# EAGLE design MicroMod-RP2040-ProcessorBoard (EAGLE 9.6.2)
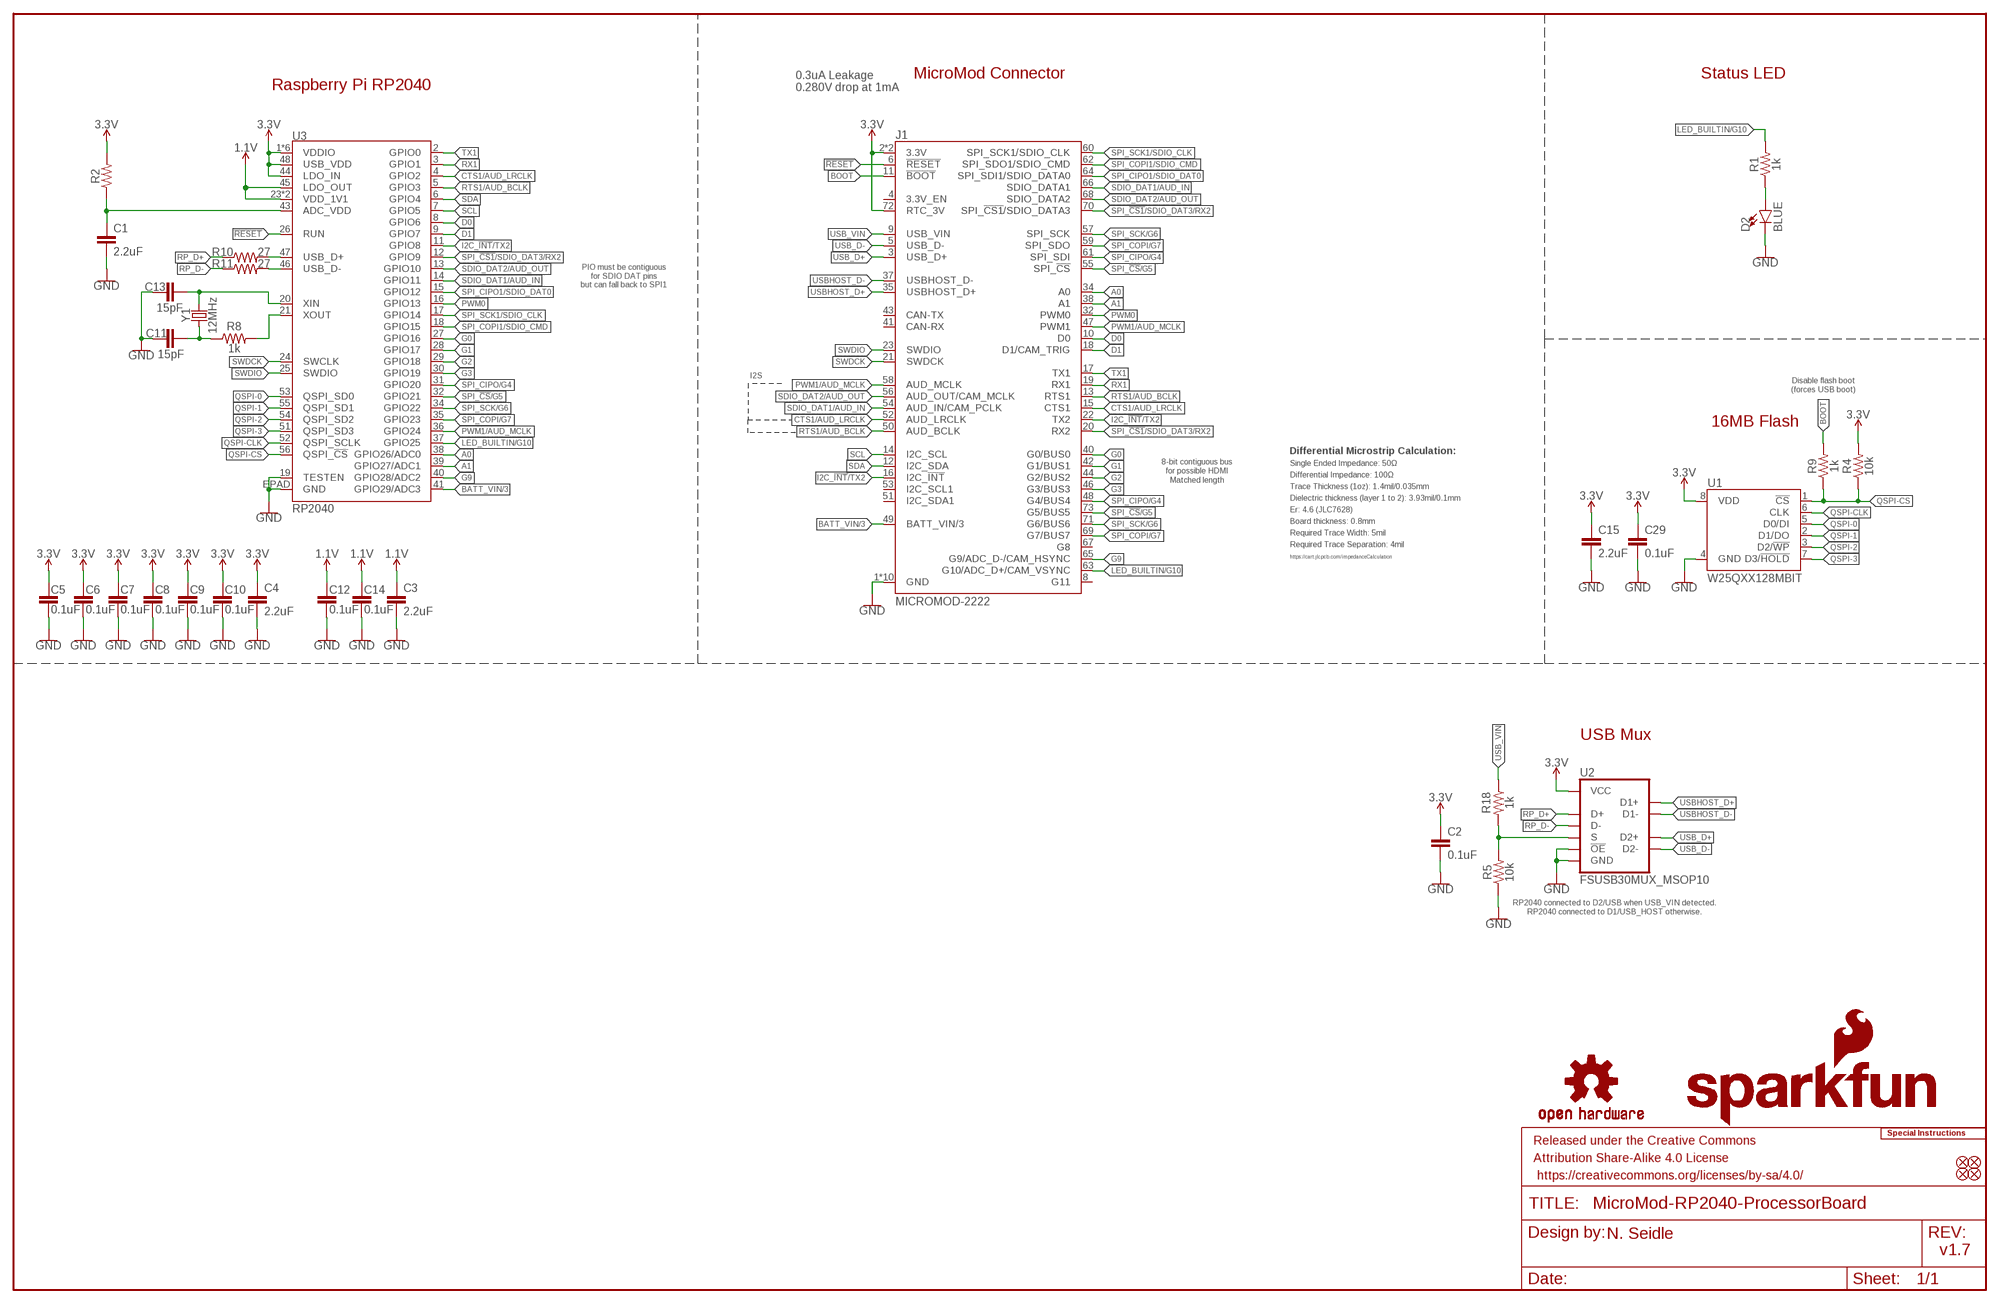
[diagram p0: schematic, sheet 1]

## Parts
C1  2.2uF  2.2UF-0402_TIGHT-10V-10%-X5R  [0402-TIGHT]
C2  0.1uF  0.1UF-0402T-6.3V-10%-X7R  [0402-TIGHT]
C3  2.2uF  2.2UF-0402_TIGHT-10V-10%-X5R  [0402-TIGHT]
C4  2.2uF  2.2UF-0402_TIGHT-10V-10%-X5R  [0402-TIGHT]
C5  0.1uF  0.1UF-0402T-6.3V-10%-X7R  [0402-TIGHT]
C6  0.1uF  0.1UF-0402T-6.3V-10%-X7R  [0402-TIGHT]
C7  0.1uF  0.1UF-0402T-6.3V-10%-X7R  [0402-TIGHT]
C8  0.1uF  0.1UF-0402T-6.3V-10%-X7R  [0402-TIGHT]
C9  0.1uF  0.1UF-0402T-6.3V-10%-X7R  [0402-TIGHT]
C10  0.1uF  0.1UF-0402T-6.3V-10%-X7R  [0402-TIGHT]
C11  15pF  15PF-0402T-50V-5%  [0402-TIGHT]
C12  0.1uF  0.1UF-0402T-6.3V-10%-X7R  [0402-TIGHT]
C13  15pF  15PF-0402T-50V-5%  [0402-TIGHT]
C14  0.1uF  0.1UF-0402T-6.3V-10%-X7R  [0402-TIGHT]
C15  2.2uF  2.2UF-0402_TIGHT-10V-10%-X5R  [0402-TIGHT]
C29  0.1uF  0.1UF-0402T-6.3V-10%-X7R  [0402-TIGHT]
D2  BLUE  LED-BLUE0603  [LED-0603]
FD1  FIDUCIALUFIDUCIAL  [FIDUCIAL-MICRO]
FD2  FIDUCIALUFIDUCIAL  [FIDUCIAL-MICRO]
FD3  FIDUCIALUFIDUCIAL  [FIDUCIAL-MICRO]
FD4  FIDUCIALUFIDUCIAL  [FIDUCIAL-MICRO]
FRAME1  FRAME-LEDGER  [CREATIVE_COMMONS]
J1  MICROMOD-2222  [M.2-CARD-E-22]
LOGO1  SFE_LOGO_NAME_FLAME.1_INCH  [SFE_LOGO_NAME_FLAME_.1]
LOGO2  SFE_LOGO_FLAME.1_INCH  [SFE_LOGO_FLAME_.1]
LOGO3  OSHW-LOGOMINI  [OSHW-LOGO-MINI]
LOGO4  SPECIAL_INSTRUCTIONS-ORDERING  [ORDERING_INSTRUCTIONS]
R1  1k  1KOHM-0402T-1/16W-1%  [0402-TIGHT]
R2  200OHM-0402T-1/16W-1%  [0402-TIGHT]
R4  10k  10KOHM-0402T-1/16W-1%  [0402-TIGHT]
R5  10k  10KOHM-0402T-1/16W-1%  [0402-TIGHT]
R8  1k  1KOHM-0402T-1/16W-1%  [0402-TIGHT]
R9  1k  1KOHM-0402T-1/16W-1%  [0402-TIGHT]
R10  27  27OHM  [0402-TIGHT]
R11  27  27OHM  [0402-TIGHT]
R18  1k  1KOHM-0402T-1/16W-1%  [0402-TIGHT]
U1  W25QXX128MBIT  W25QXX128MBIT-6X5-SKINNY_CENTER  [WSON-8-6X5-SKINNY_CENTERPAD]
U2  FSUSB30MUX_MSOP10  [MSOP10]
U3  RP2040  [QFN-56]
Y1  12MHz  CRYSTAL-12MHZ  [CRYSTAL-SMD-2X2.5MM]

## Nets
1.1V: C3.1 C12.1 C14.1 U3.23(VDD_1V1) U3.45(LDO_OUT) U3.50(VDD_1V1)
3.3V: C2.1 C4.1 C5.1 C6.1 C7.1 C8.1 C9.1 C10.1 C15.1 C29.1 J1.2(3.3V) J1.72(RTC_3V) J1.74(3.3V) R2.2 R4.2 U1.8(VDD) U2.10(VCC) U3.1(VDDIO) U3.10(VDDIO) U3.22(VDDIO) U3.33(VDDIO) U3.42(VDDIO) U3.44(LDO_IN) U3.48(USB_VDD) U3.49(VDDIO)
!RESET!: J1.6(!RESET!) U3.26(RUN)
A0: J1.34(A0) U3.38(GPIO26/ADC0)
A1: J1.38(A1) U3.39(GPIO27/ADC1)
ADC_VDD: C1.1 R2.1 U3.43(ADC_VDD)
BATT_VIN/3: J1.49(BATT_VIN/3) U3.41(GPIO29/ADC3)
BOOT: J1.11(!BOOT!) R9.2
CTS1/AUD_LRCLK: J1.15(CTS1) J1.52(AUD_LRCLK) U3.4(GPIO2)
D0: J1.10(D0) U3.8(GPIO6)
D1: J1.18(D1/CAM_TRIG) U3.9(GPIO7)
G0 [DiffPair]: J1.40(G0/BUS0) U3.27(GPIO16)
G1 [DiffPair]: J1.42(G1/BUS1) U3.28(GPIO17)
G2 [DiffPair]: J1.44(G2/BUS2) U3.29(GPIO18)
G3 [DiffPair]: J1.46(G3/BUS3) U3.30(GPIO19)
G9: J1.65(G9/ADC_D-/CAM_HSYNC) U3.40(GPIO28/ADC2)
GND: C1.2 C2.2 C3.2 C4.2 C5.2 C6.2 C7.2 C8.2 C9.2 C10.2 C11.1 C12.2 C13.1 C14.2 C15.2 C29.2 D2.C J1.1(GND) J1.7(GND) J1.33(GND) J1.36(GND) J1.39(GND) J1.45(GND) J1.75(GND) J1.GND1(GND) J1.GND2(GND) J1.GND3(GND) R5.1 U1.4(GND) U2.5(GND) U2.9(!OE!) U3.19(TESTEN) U3.EPAD(GND)
I2C_!INT!/TX2: J1.16(I2C_!INT!) J1.22(TX2) U3.11(GPIO8)
LED_BUILTIN/G10: J1.63(G10/ADC_D+/CAM_VSYNC) R1.2 U3.37(GPIO25)
N$2: D2.A R1.1
N$4: R8.2 U3.21(XOUT)
N$5: C13.2 U3.20(XIN) Y1.P3
N$6: C11.2 R8.1 Y1.P1
PWM0: J1.32(PWM0) U3.16(GPIO13)
PWM1/AUD_MCLK: J1.47(PWM1) J1.58(AUD_MCLK) U3.36(GPIO24)
QSPI-0: U1.5(D0/DI) U3.53(QSPI_SD0)
QSPI-1: U1.2(D1/DO) U3.55(QSPI_SD1)
QSPI-2: U1.3(D2/!WP!) U3.54(QSPI_SD2)
QSPI-3: U1.7(D3/!HOLD!) U3.51(QSPI_SD3)
QSPI-CLK [Clock]: U1.6(CLK) U3.52(QSPI_SCLK)
QSPI-CS: R4.1 R9.1 U1.1(!CS!) U3.56(QSPI_!CS!)
RP_D1+: R10.2 U3.47(USB_D+)
RP_D1-: R11.2 U3.46(USB_D-)
RP_D+: R10.1 U2.4(D+)
RP_D-: R11.1 U2.6(D-)
RTS1/AUD_BCLK: J1.13(RTS1) J1.50(AUD_BCLK) U3.5(GPIO3)
RX1: J1.19(RX1) U3.3(GPIO1)
SCL: J1.14(I2C_SCL) U3.7(GPIO5)
SDA: J1.12(I2C_SDA) U3.6(GPIO4)
SDIO_DAT1/AUD_IN: J1.54(AUD_IN/CAM_PCLK) J1.66(SDIO_DATA1) U3.14(GPIO11)
SDIO_DAT2/AUD_OUT: J1.56(AUD_OUT/CAM_MCLK) J1.68(SDIO_DATA2) U3.13(GPIO10)
SPI_!CS1!/SDIO_DAT3/RX2: J1.20(RX2) J1.70(SPI_!CS1!/SDIO_DATA3) U3.12(GPIO9)
SPI_!CS!/G5 [DiffPair]: J1.55(SPI_!CS!) J1.73(G5/BUS5) U3.32(GPIO21)
SPI_CIPO1/SDIO_DAT0: J1.64(SPI_SDI1/SDIO_DATA0) U3.15(GPIO12)
SPI_CIPO/G4 [DiffPair]: J1.48(G4/BUS4) J1.61(SPI_SDI) U3.31(GPIO20)
SPI_COPI1/SDIO_CMD: J1.62(SPI_SDO1/SDIO_CMD) U3.18(GPIO15)
SPI_COPI/G7 [DiffPair]: J1.59(SPI_SDO) J1.69(G7/BUS7) U3.35(GPIO23)
SPI_SCK1/SDIO_CLK: J1.60(SPI_SCK1/SDIO_CLK) U3.17(GPIO14)
SPI_SCK/G6 [DiffPair]: J1.57(SPI_SCK) J1.71(G6/BUS6) U3.34(GPIO22)
SWDCK: J1.21(SWDCK) U3.24(SWCLK)
SWDIO: J1.23(SWDIO) U3.25(SWDIO)
TX1: J1.17(TX1) U3.2(GPIO0)
USB_D+: J1.3(USB_D+) U2.3(D2+)
USB_D-: J1.5(USB_D-) U2.7(D2-)
USB_MUX_SIG: R5.2 R18.2 U2.1(S)
USB_VIN: J1.9(USB_VIN) R18.1
USBHOST_D+: J1.35(USBHOST_D+) U2.2(D1+)
USBHOST_D-: J1.37(USBHOST_D-) U2.8(D1-)
Unconnected: J1.4(3.3V_EN) J1.8(G11) J1.41(CAN-RX) J1.43(CAN-TX) J1.51(I2C_SDA1) J1.53(I2C_SCL1) J1.67(G8)

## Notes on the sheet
- MicroMod Connector | Status LED
- Raspberry Pi RP2040
- 0.3uA Leakage
  0.280V drop at 1mA
- PIO must be contiguous
  for SDIO DAT pins
  but can fall back to SPI1
- I2S
- Disable flash boot
  (forces USB boot)
- 16MB Flash
- Differential Microstrip Calculation:
- 8-bit contiguous bus
  for possible HDMI
- Single Ended Impedance: 50Ω
- Differential Impedance: 100Ω
- Matched length
- Trace Thickness (1oz): 1.4mil/0.035mm
- Dielectric thickness (layer 1 to 2): 3.93mil/0.1mm
- Er: 4.6 (JLC7628)
- Board thickness: 0.8mm
- Required Trace Width: 5mil
- Required Trace Separation: 4mil
- https://cart.jlcpcb.com/impedanceCalculation
- USB Mux
- RP2040 connected to D2/USB when USB_VIN detected.
  RP2040 connected to D1/USB_HOST otherwise.
- N. Seidle
- v1.7

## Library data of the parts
C1 C3 C4 C15 = SparkFun-Capacitors:2.2UF: 2.2µF ceramic capacitors; PROD_ID: CAP-14232
C2 C5-C10 C12 C14 C29 = SparkFun-Capacitors:0.1UF: 0.1µF ceramic capacitors; PROD_ID: CAP-14993
C11 C13 = SparkFun-Capacitors:15PF: 15pF ceramic capacitors; PROD_ID: CAP-13063
D2 = SparkFun-LED:LED-BLUE: Blue SMD LED; PROD_ID: DIO-08575
FD1-FD4 = SparkFun-Aesthetics:FIDUCIAL: Fiducial Alignment Points
FRAME1 = SparkFun-Aesthetics:FRAME-LEDGER: Schematic Frame - Ledger
J1 = SparkFun-MicroMod:MICROMOD: MicroMod Connector Description: A card edge connector and mating PCB connector to allow various MicroMod Processor Boards to be coupled with various carrier boards of different capabilities. Based on the M.2 standard.
LOGO1 = SparkFun-Aesthetics:SFE_LOGO_NAME_FLAME: SparkFun Font Logo w/ Flame
LOGO2 = SparkFun-Aesthetics:SFE_LOGO_FLAME: SparkFun Flame Logo
LOGO3 = SparkFun-Aesthetics:OSHW-LOGO: Open-Source Hardware (OSHW) Logo
LOGO4 = SparkFun-Aesthetics:SPECIAL_INSTRUCTIONS: Special Ordering/Production Instructions Alert
R1 R8 R9 R18 = SparkFun-Resistors:1KOHM: 1kΩ resistor; PROD_ID: RES-14342
R2 = SparkFun-Resistors:200OHM: 200Ω resistor; PROD_ID: RES-15550
R4 R5 = SparkFun-Resistors:10KOHM: 10kΩ resistor; PROD_ID: RES-14241
R10 R11 = SparkFun-Resistors:27OHM: 27Ω resistor; PROD_ID: RES-15238
U1 = SparkFun-IC-Memory:W25QXX; PROD_ID: IC-15107
U2 = SparkFun-IC-Special-Function:FSUSB30MUX; PROD_ID: IC-15569
U3 = RP2040:RP2040: Raspberry Pi RP2040 MCU 56-pin 32-bit Microcontroller with 264kB of SRAM and external flash support up to 16MB Getting Started with the RP2040 Dual-core ARM Cortex M0+ processor, flexible clock running up to 133 MHz 264kB of SRAM, and QSPI control of common flash memory USB 1.1 Host and Device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; PROD_ID: IC-15502
Y1 = SparkFun-Clocks:CRYSTAL-12MHZ: 12.0MHz Crystal; PROD_ID: XTAL-15540

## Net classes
1 DiffPair: width 0.127 mm, clearance 0.178 mm
2 Clock: width 0.089 mm, clearance 0.178 mm
4 InternalPower: width 0.152 mm

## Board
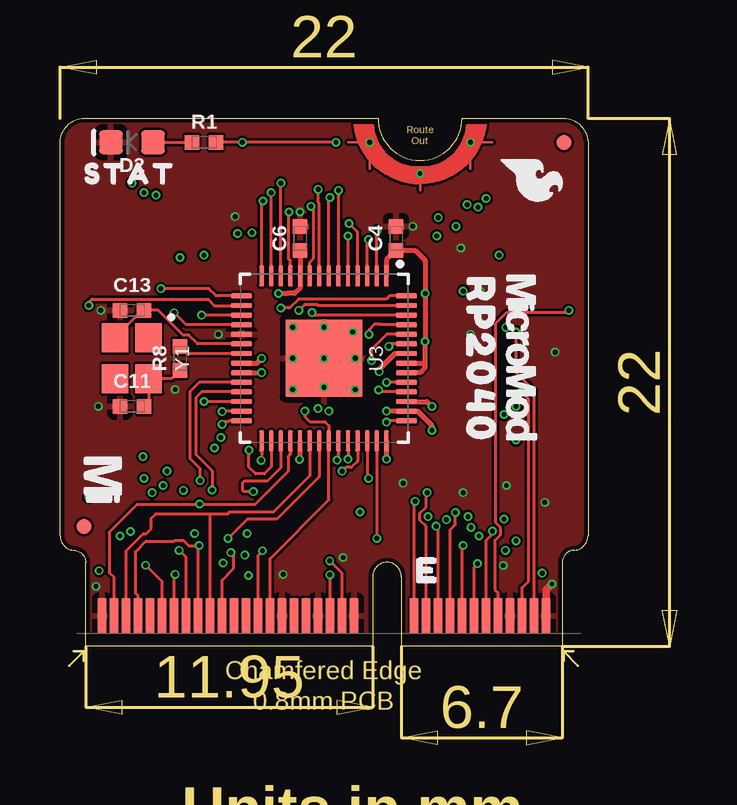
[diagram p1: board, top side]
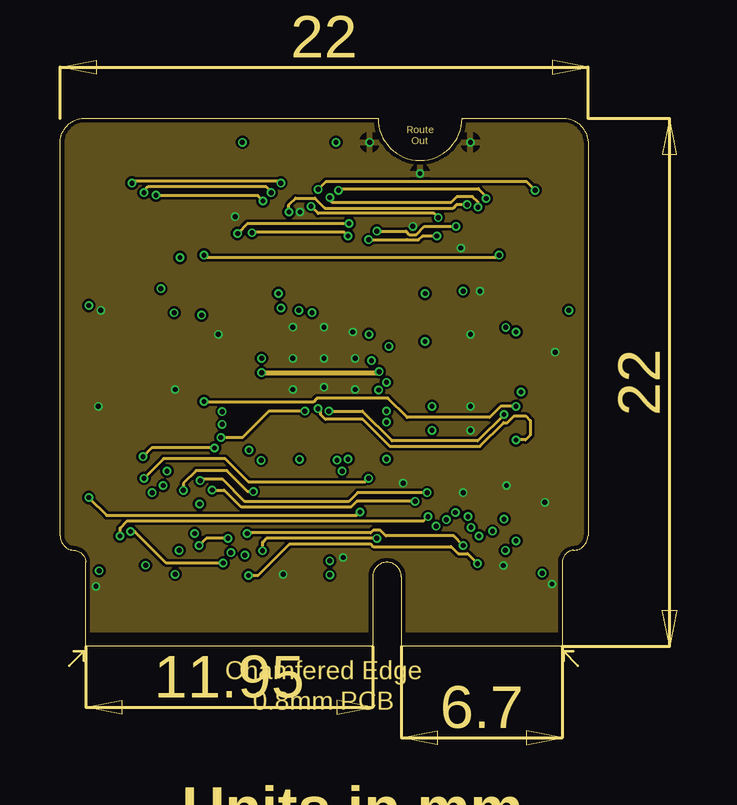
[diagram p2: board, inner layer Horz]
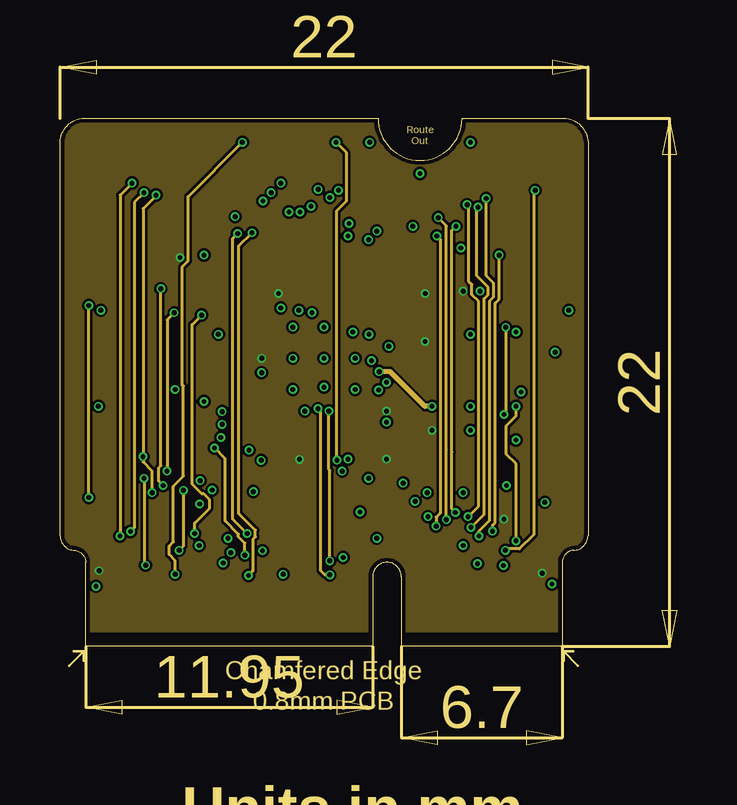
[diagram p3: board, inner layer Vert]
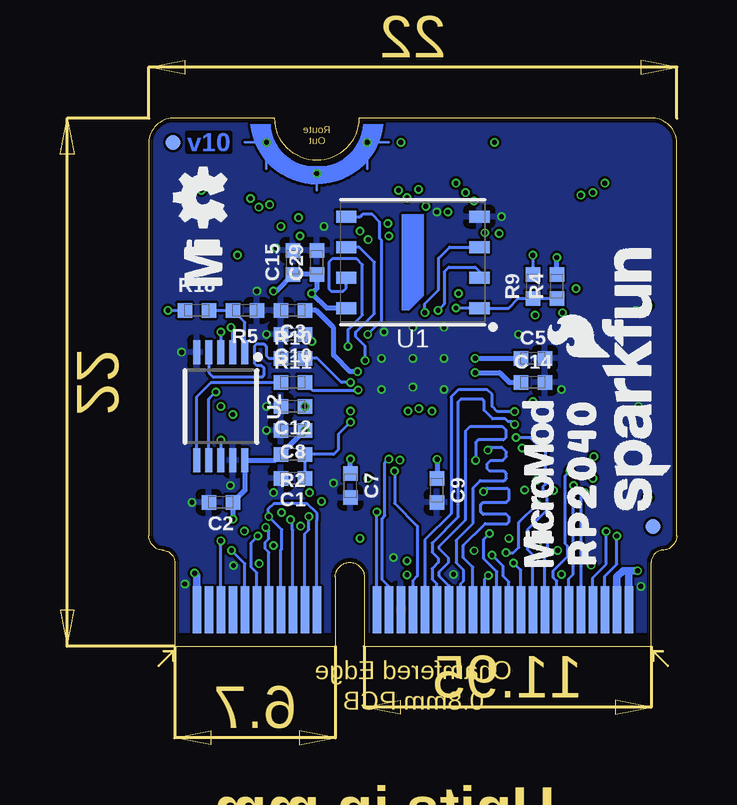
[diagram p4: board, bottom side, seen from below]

Size 25.7 x 28.54 mm. Coordinates in mm from the lower left corner, seen from the top.
Outline: 0,8.71 0,25.11 arc-87 1,26.11 13.25,26.11 arc180 16.75,26.11 21,26.11 arc-87 22,25.11 22,8.71
Outline: 0,8.71 arc87 0.6,8.11
Outline: 21.4,8.11 arc87 22,8.71
Outline: 21.4,8.11 arc85 20.93,7.61 20.93,4.11 14.22,4.11 14.22,7.01 arc180 13.03,7.01 13.03,4.11 1.07,4.11 1.07,7.61 arc84 0.6,8.11
Outline: 21.4,8.11 arc87 22,8.71
Outline: 0,8.71 arc87 0.6,8.11
Copper layers (1+2*15+16): Top 0.035mm / dielectric 1.5mm / Horz 0.035mm / dielectric 0.15mm / Vert 0.035mm / dielectric 0.2mm / Bottom 0.035mm
Design rules "SparkFun-4-layer-MicroMod": minimum track width 4mil, minimum drill 0.2mm, track to track 4mil, track to pad 4mil, pad to pad 4mil, via to via 4mil, smd to smd 4mil, copper to edge 6mil, drill to drill 6mil, minimum pad ring 3mil, minimum via ring 3mil, stop-mask expansion 4mil, vias tented up to drill 25mil, thermal gap 10mil

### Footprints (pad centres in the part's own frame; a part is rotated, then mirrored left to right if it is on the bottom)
0402-TIGHT = smd 0.6 x 0.6: 1 -0.5,0; 2 0.5,0
LED-0603 = smd 1 x 1: A -0.877,0; C 0.877,0
FIDUCIAL-MICRO = smd 0.635 x 0.635: 1 0,0
M.2-CARD-E-22 = smd 0.35 x 1.45: 1 9.25,1.275; 3 8.75,1.275; 5 8.25,1.275; 7 7.75,1.275; 9 7.25,1.275; 11 6.75,1.275; 13 6.25,1.275; 15 5.75,1.275; 17 5.25,1.275; 19 4.75,1.275; 21 4.25,1.275; 23 3.75,1.275; 33 1.25,1.275; 35 0.75,1.275; 37 0.25,1.275; 39 -0.25,1.275; 41 -0.75,1.275; 43 -1.25,1.275; 45 -1.75,1.275; 47 -2.25,1.275; 49 -2.75,1.275; 51 -3.25,1.275; 53 -3.75,1.275; 55 -4.25,1.275; 57 -4.75,1.275; 59 -5.25,1.275; 61 -5.75,1.275; 63 -6.25,1.275; 65 -6.75,1.275; 67 -7.25,1.275; 69 -7.75,1.275; 71 -8.25,1.275; 73 -8.75,1.275; 75 -9.25,1.275 | smd 0.35 x 1.95 bottom: 2 9,1.525; 4 8.5,1.525; 6 8,1.525; 8 7.5,1.525; 10 7,1.525; 12 6.5,1.525; 14 6,1.525; 16 5.5,1.525; 18 5,1.525; 20 4.5,1.525; 22 4,1.525; 32 1.5,1.525; 34 1,1.525; 36 0.5,1.525; 38 0,1.525; 40 -0.5,1.525; 42 -1,1.525; 44 -1.5,1.525; 46 -2,1.525; 48 -2.5,1.525; 50 -3,1.525; 52 -3.5,1.525; 54 -4,1.525; 56 -4.5,1.525; 58 -5,1.525; 60 -5.5,1.525; 62 -6,1.525; 64 -6.5,1.525; 66 -7,1.525; 68 -7.5,1.525; 70 -8,1.525; 72 -8.5,1.525; 74 -9,1.525 | drill 0.2: GND1 1.9,21; GND2 4,19.7; GND3 6.1,21
WSON-8-6X5-SKINNY_CENTERPAD = smd 0.85 x 0.5: 1 -2.775,1.905; 2 -2.775,0.635; 3 -2.775,-0.635; 4 -2.775,-1.905; 5 2.775,-1.905; 6 2.775,-0.635; 7 2.775,0.635; 8 2.775,1.905
MSOP10 = smd 1 x 0.3: 1 -2.25,1; 2 -2.25,0.5; 3 -2.25,0; 4 -2.25,-0.5; 5 -2.25,-1; 6 2.25,-1; 7 2.25,-0.5; 8 2.25,0; 9 2.25,0.5; 10 2.25,1
QFN-56 = smd 0.875 x 0.2: 1 -3.437,2.6; 2 -3.437,2.2; 3 -3.437,1.8; 4 -3.437,1.4; 5 -3.437,1; 6 -3.437,0.6; 7 -3.437,0.2; 8 -3.437,-0.2; 9 -3.437,-0.6; 10 -3.437,-1; 11 -3.437,-1.4; 12 -3.437,-1.8; 13 -3.437,-2.2; 14 -3.437,-2.6; 29 3.437,-2.6; 30 3.437,-2.2; 31 3.437,-1.8; 32 3.437,-1.4; 33 3.437,-1; 34 3.437,-0.6; 35 3.437,-0.2; 36 3.437,0.2; 37 3.437,0.6; 38 3.437,1; 39 3.437,1.4; 40 3.437,1.8; 41 3.437,2.2; 42 3.437,2.6 | smd 0.2 x 0.875: 15 -2.6,-3.437; 16 -2.2,-3.437; 17 -1.8,-3.437; 18 -1.4,-3.437; 19 -1,-3.437; 20 -0.6,-3.437; 21 -0.2,-3.437; 22 0.2,-3.437; 23 0.6,-3.437; 24 1,-3.437; 25 1.4,-3.437; 26 1.8,-3.437; 27 2.2,-3.437; 28 2.6,-3.437; 43 2.6,3.437; 44 2.2,3.437; 45 1.8,3.437; 46 1.4,3.437; 47 1,3.437; 48 0.6,3.437; 49 0.2,3.437; 50 -0.2,3.437; 51 -0.6,3.437; 52 -1,3.437; 53 -1.4,3.437; 54 -1.8,3.437; 55 -2.2,3.437; 56 -2.6,3.437 | smd 3.2 x 3.2: EPAD 0,0
CRYSTAL-SMD-2X2.5MM = smd 1.2 x 1.1: P1 0.846,0.69; P2 -0.854,0.69; P3 -0.854,-0.71; P4 0.846,-0.71

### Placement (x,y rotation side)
C1  16,11.11 180 bottom
C2  19,10.11 180 bottom
C3  16,18.11 180 bottom
C4  14,21.11 90 top
C5  6,16.11 0 bottom
C6  10,21.11 90 top
C7  13.6,10.81 270 bottom
C8  16,13.11 180 bottom
C9  10,10.61 270 bottom
C10  16,17.11 180 bottom
C11  3,14.11 0 top
C12  16,14.11 180 bottom
C13  3,18.11 0 top
C14  6,15.11 0 bottom
C15  16,20.11 90 bottom
C29  15,20.11 90 bottom
D2  3,25.11 180 top
FD1  1,9.11 0 top
FD2  21,25.11 0 top
FD3  21,25.11 0 bottom
FD4  1,9.11 0 bottom
FRAME1  not placed on the board
J1  11,4.11 0 top
LOGO1  1.7,15.31 90 bottom
LOGO2  19.68,23.54 270 top
LOGO3  19.75,22.81 90 bottom
LOGO4  not placed on the board
R1  6,25.11 0 top
R2  16,12.11 180 bottom
R4  5,19.11 90 bottom
R5  18,18.11 180 bottom
R8  5,16.11 90 top
R9  6,19.11 90 bottom
R10  16,16.11 0 bottom
R11  16,15.11 0 bottom
R18  20,18.11 0 bottom
U1  11,20.11 180 bottom
U2  19,14.11 270 bottom
U3  11,16.11 270 top
U$1  [MICROMOD_MI_LOGO_.35]  1.81,11.08 270 top
U$3  [MICROMOD_LOGO_.3]  5.71,10.84 90 bottom
U$4  [RP20400]  3.94,10.97 90 bottom
U$7  [MICROMOD_MI_LOGO_.35]  19.75,20.07 90 bottom
U$9  [RP20400]  17.53,16.05 270 top
U$11  [STAT0]  0.38,23.79 0 top
U$12  [MICROMOD_LOGO_.3]  19.18,16.18 270 top
Y1  3,16.11 270 top

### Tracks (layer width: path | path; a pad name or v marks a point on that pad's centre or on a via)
1.1V  (via drill 0.2)
  Top 0.203: U3.45 15.3,14.31 C12.1 | U3.50 13.95,16.31 13.3,15.66 v13.3,15.56 | U3.23 v8.4,15.51
  Horz 0.127: v13.3,15.56 13.3,15.51
  Horz 0.203: v8.4,15.51 13.3,15.51
  Vert 0.203: C12.1 15.2,14.11 13.75,15.56 v13.3,15.56
  Bottom 0.203: v8.4,15.51 7.38,15.51 6.98,15.11 C14.1 | v13.3,15.56 13.62,15.56 14.3,16.23 14.3,17.38 15.03,18.11 C3.1
  other vias: 15.5,14.11
3.3V  (via drill 0.2)
  Top 0.127: v15.21,16.81 v15.21,16.82
  Top 0.203: U3.42 v13.6,11.91 | v13.6,13.91 U3.44 14.9,13.91 15.5,13.31 C8.1 | U3.48 15,15.51 15.21,15.72 15.21,15.91 | v9.98,11.9 10,11.92 U3.33 | C6.1 U3.10 10,19.04 9.77,18.81 9.48,18.81 v9.1,18.81 | U3.1 13.6,20.21 C4.1 14.8,20.61 15.21,20.2 v15.21,18.81 v15.21,16.82 | v15.21,16.81 15.21,15.91 | U3.49 15.21,15.91 | U3.22 8.2,15.91 v8.4,16.11
  Bottom 0.127: v15.21,16.82 v15.21,16.81 | C9.1 9.98,11.13 | 15.18,18.81 v15.21,18.81
  Bottom 0.203: C10.1 v15.21,16.82 | v9.98,11.9 9.98,11.13 | R4.2 v5,20.31 | v18.5,9.41 C2.1 18,10.61 U2.10 16.75,11.86 R2.2 C8.1 | C7.1 v13.6,11.91 | v16.8,18.91 16.7,18.91 C15.1 C29.1 15,19.02 v15.21,18.81 | 15.18,18.81 14.57,18.21 U1.8 | v8.4,16.11 C5.1
  Bottom 0.305: J1.72 2.5,7 2.24,7.26 v1.63,7.26 1.93,7.26 2,7.19 J1.74 | J1.2 20,7.07 v20.09,7.16
  other vias: 15.5,13.11
  pour Vert (isolate 0.102): 0,26.11 22,26.11 22,4.75 0,4.75
!RESET!  (via drill 0.2)
  Top 0.127: U3.26 v6,14.31
  Horz 0.127: v6,14.31 10.56,14.31 10.71,14.45 13.66,14.45 14.46,13.65 17.9,13.65 18.36,14.11 v19,14.11
  Vert 0.127: v19,8.51 19,11.71 18.6,12.11 18.6,13.31 19,13.71 v19,14.11
  Bottom 0.127: J1.6 v19,8.51
A0  (via drill 0.2)
  Top 0.127: U3.38 v12,11.91
  Bottom 0.127: J1.34 12,6.61 12.27,6.88 12.27,9.46 12.16,9.57 12.16,11.75 v12,11.91
A1  (via drill 0.2)
  Top 0.127: v11.76,11.41 11.92,11.57 12.14,11.57 12.4,11.83 U3.39
  Bottom 0.127: v11.76,11.41 11.76,10.07 10.8,9.12 10.8,7.04 11,6.85 J1.38
ADC_VDD  (via drill 0.2)
  Top 0.127: U3.43 13.66,13.51 v13.6,13.45
  Bottom 0.127: v13.6,13.45 14.1,12.95 14.1,12.31 14.3,12.11 R2.1 C1.1
BATT_VIN/3  (via drill 0.2)
  Top 0.127: U3.41 v13.2,8.61 | v8.44,8.09 8.25,7.9 J1.49
  Horz 0.127: v13.2,8.61 8.6,8.61 8.44,8.45 v8.44,8.09
BOOT  (via drill 0.2)
  Top 0.127: J1.11 17.75,8.52 18.02,8.79 v18.02,8.91
  Horz 0.127: v18.3,20.41 18.2,20.31 6.1,20.31 v6,20.41
  Vert 0.127: v18.02,8.91 18.02,9.16 18.13,9.26 18.13,18.41 18.3,18.58 v18.3,20.41
  Bottom 0.127: v6,20.41 R9.2
CTS1/AUD_LRCLK  (via drill 0.2)
  Top 0.127: U3.4 12.4,21.37 v12.04,21.73 | J1.15 16.75,8.26 v16.8,8.31
  Horz 0.127: v12.04,21.73 7.82,21.73 v7.4,21.31 | v16.8,8.31 16.4,8.71 13.58,8.71 13.34,8.95 13.06,8.95 12.95,8.84 7.83,8.84 v7.8,8.81
  Vert 0.127: v7.4,21.31 7.2,21.11 7.2,9.41 v7.8,8.81
  Bottom 0.127: J1.52 7.5,7.23 8.04,7.77 8.04,8.57 v7.8,8.81
D0  (via drill 0.2)
  Top 0.127: U3.8 10.8,22.58 10.76,22.62 v10.76,23.15
  Horz 0.127: v10.76,23.15 11.08,23.47 19.44,23.47 v19.8,23.11
  Vert 0.127: v18.56,8.11 18.61,8.17 19.14,8.17 19.75,8.77 19.75,23.06 v19.8,23.11
  Bottom 0.127: J1.10 18,7.55 v18.56,8.11
D1  (via drill 0.2)
  Top 0.127: U3.9 10.4,20.11 10.57,20.28 10.57,22.33 v10.46,22.44
  Horz 0.127: v10.46,22.44 10.76,22.14 15.59,22.14 v15.76,21.97
  Vert 0.127: v16.09,9.39 16.09,12.3 16.1,12.31 16.1,21.63 v15.76,21.97
  Bottom 0.127: v16.09,9.39 16.01,9.31 16.01,8.97 16,8.96 J1.18
G0  (via drill 0.2)
  Top 0.127: U3.27 6.78,13.91 v6.76,13.89
  Bottom 0.127: J1.40 10.5,8.54 9.4,9.64 9.4,14.5 9.11,14.8 7.9,14.8 7.7,14.61 7.7,14.11 7.48,13.89 v6.76,13.89
G1  (via drill 0.2)
  Top 0.127: U3.28 7.07,13.51 7.03,13.47 6.87,13.47 v6.76,13.36
  Bottom 0.127: v6.76,13.36 6.87,13.47 7.03,13.47 7.14,13.58 7.67,13.58 8.03,13.94 8.03,14.34 8.1,14.41 9,14.41 9.1,14.31 9.1,9.51 10.2,8.41 10.2,8.04 9.93,7.78 9.93,7.61 10.2,7.35 10.2,6.91 10,6.71 J1.42
G2  (via drill 0.2)
  Top 0.127: v8.38,11.86 8.4,11.88 U3.29
  Bottom 0.127: J1.44 9.5,6.64 9.89,7.03 9.89,7.22 9.51,7.61 9.51,7.78 9.89,8.17 9.89,8.29 8.79,9.38 8.79,13.08 8.6,13.28 7.27,13.28 7.12,13.13 7.12,12.81 7.22,12.71 8.27,12.71 8.38,12.59 v8.38,11.86
G3  (via drill 0.2)
  Top 0.127: v7.87,12.28 7.87,11.58 8.15,11.3 8.51,11.3 8.8,11.59 U3.30
  Bottom 0.127: J1.46 9,6.72 8.88,6.84 8.88,7.28 9.2,7.6 9.2,8.53 8.48,9.24 8.48,10.72 8.19,11.01 7.2,11.01 7.1,11.11 7.1,11.31 7.2,11.41 7.8,11.41 7.9,11.51 7.9,11.71 7.75,11.86 7.25,11.86 7.1,12.01 7.1,12.21 7.29,12.41 7.75,12.41 v7.87,12.28
G9  (via drill 0.2)
  Top 0.127: U3.40 12.8,11.17 v12.86,11.11 | J1.65 4.25,6.81 v3.57,7.49
  Horz 0.127: v3.5,11.11 4.32,11.93 6.88,11.93 7.83,10.97 12.72,10.97 v12.86,11.11
  Vert 0.127: v3.5,11.11 3.5,7.56 v3.57,7.49
GND  (via drill 0.2)
  Top 0.305: J1.1 20.25,6.46 v20.5,6.71
  other vias: 18.47,7.48 16.8,10.51 17.1,13.11 18.6,10.81 17.1,14.11 20.63,16.37 16.7,20.71 14.7,21.61 7.3,22.01 6.6,17.11 14.3,10.91 9.7,17.41 12.2,17.21 12.3,14.81 9.7,14.81 11,16.11 1.6,14.11 1.7,18.11 4.8,14.81 17.5,18.91 17.1,17.11 11.8,7.81 9.3,7.11 1.5,6.61 10,22.21 9.7,16.11 12.3,16.11 11,14.91 11,17.41 20.2,10.11
  pour Top (isolate 0.102): 0,26.11 22,26.11 22,4.71 0,4.71
  pour Bottom (isolate 0.102): 0,26.11 22,26.11 22,4.71 0,4.71
  pour Horz (isolate 0.102): 0,4.75 0,26.11 22,26.11 22,4.75
I2C_!INT!/TX2  (via drill 0.2)
  Top 0.127: U3.11 9.6,20.18 9.54,20.24 v9.54,22.2 v9.54,22.21
  Horz 0.127: v9.54,22.21 9.54,22.51 9.82,22.79 10.62,22.79 11.04,22.37 16.38,22.37 16.52,22.51 v16.96,22.51
  Vert 0.127: v17,9.51 17.44,9.95 17.44,18.49 17.16,18.77 17.16,19.19 17.04,19.3 17.04,22.43 v16.96,22.51
  Bottom 0.127: J1.16 16.5,8.13 16.46,8.17 16.46,8.97 v17,9.51 17.04,9.55 17.04,9.81 16.79,10.06 15.4,10.06 14.99,9.65 14.99,9.37 15,9.36 J1.22
LED_BUILTIN/G10  (via drill 0.2)
  Top 0.127: U3.37 11.6,11.92 v11.54,11.86 | v11.5,25.11 v7.6,25.11 R1.2 | J1.63 4.75,7.06 v4.8,7.11
  Vert 0.127: v11.54,11.86 11.54,22.27 11.94,22.67 11.94,24.67 v11.5,25.11 | v4.8,7.11 4.8,7.69 4.55,7.94 4.55,8.28 4.72,8.46 4.72,10.78 5.14,11.2 5.14,14.95 5.1,14.99 5.1,19.93 5.34,20.17 5.34,22.85 v7.6,25.11
N$2
  Top 0.127: D2.A R1.1
N$4
  Top 0.127: U3.21 5.3,16.31 R8.2
N$5
  Top 0.127: Y1.P3 3.44,18.11 C13.2 4.1,18.11 5.13,17.07 5.37,17.07 5.73,16.71 U3.20
N$6
  Top 0.127: R8.1 4.65,15.26 Y1.P1 3.69,14.3 C11.2
PWM0  (via drill 0.2)
  Top 0.127: U3.16 6.43,18.31 6.17,18.57 1.33,18.57 1.2,18.44 v1.2,18.31
  Horz 0.127: v1.2,10.31 1.95,9.56 12.35,9.56 v12.5,9.71
  Vert 0.127: v1.2,10.31 v1.2,18.31
  Bottom 0.127: J1.32 v12.5,9.71
PWM1/AUD_MCLK  (via drill 0.2)
  Top 0.127: J1.47 8.75,7.77 11.2,10.22 U3.36 11.2,13.31 11.04,13.47 10.4,13.47 10.2,13.67 v10.2,13.91
  Horz 0.127: v10.2,13.91 8.7,13.91 7.6,12.81 v6.7,12.81
  Bottom 0.127: v6.7,12.81 6.1,12.81 5.46,12.17 5.46,10.88 5.56,10.78 5.56,10.44 5.4,10.28 5.4,9.8 6.22,8.98 6.22,8.14 6,7.92 J1.58
QSPI-0  (via drill 0.2)
  Top 0.127: U3.53 13.37,17.51 13.36,17.53 13.1,17.53 12.88,17.31 v12.88,17.11
  Bottom 0.127: U1.5 13.2,22.02 13.1,22.11 12.7,22.11 12.38,21.79 12.38,21.11 12.3,21.03 12.3,17.69 v12.88,17.11
QSPI-1  (via drill 0.2)
  Top 0.127: U3.55 10.76,18.31 10.72,18.35 10.2,18.35 v9.95,18.11
  Bottom 0.127: U1.2 8.22,19.73 8.4,19.91 9.5,19.91 9.7,19.71 9.7,18.36 v9.95,18.11
QSPI-2  (via drill 0.2)
  Top 0.127: U3.54 10.6,17.91 v10.5,18.01
  Bottom 0.127: v10.5,18.01 10.5,18.39 9.93,18.96 9.93,20.28 9.46,20.75 U1.3
QSPI-3  (via drill 0.2)
  Top 0.127: U3.51 13.8,16.71 v13.7,16.61
  Bottom 0.127: v13.7,16.61 13.7,17.31 13.1,17.91 13.1,20.01 13.34,20.25 14.36,20.25 14.5,20.11 14.5,19.01 14.4,18.91 13.9,18.91 13.78,19.04 U1.7
QSPI-CLK  (via drill 0.2)
  Top 0.127: U3.52 13.61,17.11 12.98,16.48 v12.98,16.01
  Bottom 0.127: v12.98,16.01 12.98,16.61 13.38,17.01 13.38,17.2 12.61,17.97 12.61,20.11 13.23,20.75 U1.6
QSPI-CS  (via drill 0.2)
  Top 0.127: v9.2,18.21 9.57,18.21 9.94,18.58 13.61,18.58 13.74,18.71 U3.56
  Bottom 0.127: R4.1 R9.1 6.6,18.61 7,18.21 U1.1 v9.2,18.21
RP_D1+  (via drill 0.2)
  Top 0.127: U3.47 v13.6,15.11
  Bottom 0.127: v13.6,15.11 13.98,15.11 14.98,16.11 R10.2
RP_D1-  (via drill 0.2)
  Top 0.127: U3.46 13.36,14.71 v13.28,14.79
  Bottom 0.127: v13.28,14.79 13.44,14.79 13.46,14.77 15.16,14.77 R11.2
RP_D+
  Bottom 0.127: U2.4 19.5,15.51 19.33,15.34 17.27,15.34 17.2,15.41 17.2,15.71 17.3,15.81 17.5,15.81 17.6,15.91 17.6,16.61 17.5,16.71 17.2,16.71 17.1,16.61 17.1,16.21 17,16.11 R10.1
RP_D-
  Bottom 0.127: U2.6 20,14.51 19.4,15.11 R11.1
RTS1/AUD_BCLK  (via drill 0.2)
  Top 0.127: U3.5 v12,21.21 | J1.13 17.25,7.4 v17.4,7.55
  Horz 0.127: v12,21.21 11.84,21.37 8.03,21.37 v8,21.34 | v17.4,7.55 16.98,7.97 16.6,7.97 16.3,8.27 13.06,8.27 12.95,8.38 9.57,8.38 8.26,7.07 v7.86,7.07
  Vert 0.127: v7.86,7.07 8.04,7.25 8.04,8.57 8.14,8.67 8.14,8.95 7.45,9.64 7.45,20.8 v8,21.34
  Bottom 0.127: J1.50 8,6.92 v7.86,7.07
RX1  (via drill 0.2)
  Top 0.127: U3.3 12.8,20.99 v12.86,21.05 | J1.19 15.75,9.04 v15.67,9.12
  Horz 0.127: v15.7,21.21 15.11,21.21 14.94,21.04 14.46,21.04 14.45,21.05 v12.86,21.05
  Vert 0.127: v15.7,21.21 15.84,21.07 15.84,9.66 15.67,9.5 v15.67,9.12
SCL  (via drill 0.2)
  Top 0.127: v11.24,22.81 11.2,22.77 U3.7
  Horz 0.127: v17.42,22.41 17.42,22.62 17.18,22.85 16.54,22.85 16.29,22.6 11.35,22.6 11.24,22.71 v11.24,22.81
  Vert 0.127: v17.13,9.07 17.67,9.61 17.67,18.6 17.84,18.77 17.84,19.07 17.37,19.54 17.37,22.36 v17.42,22.41
  Bottom 0.127: v17.13,9.07 17,8.94 17,8.59 17.14,8.45 17.14,8.17 17,8.03 J1.14
SDA  (via drill 0.2)
  Top 0.127: v11.6,23.11 U3.6
  Horz 0.127: v17.76,22.77 17.76,22.85 17.43,23.18 11.67,23.18 v11.6,23.11
  Vert 0.127: v17.45,8.71 17.45,8.91 17.9,9.36 17.9,18.5 18.07,18.67 18.07,19.24 17.76,19.55 v17.76,22.77
  Bottom 0.127: J1.12 17.5,7.17 17.74,7.41 17.74,8.42 v17.45,8.71
SDIO_DAT1/AUD_IN  (via drill 0.2)
  Top 0.127: U3.14 8.4,22.61 v8.46,22.67
  Horz 0.127: v8.46,22.67 8.24,22.88 4.03,22.88 v4,22.91 | v6.44,12.37 3.82,12.37 v3.46,12.01
  Vert 0.127: v4,22.91 4,22.89 3.46,22.35 v3.46,12.01 3.46,11.79 3.84,11.41 v3.84,10.51 | v7.7,7.91 7.7,8.41 7.43,8.68 7.43,8.79 6.88,9.34 6.88,11.93 v6.44,12.37
  Bottom 0.127: J1.54 7,6.8 7.24,7.04 7.24,7.45 v7.7,7.91 | v3.84,10.51 4,10.35 J1.66
SDIO_DAT2/AUD_OUT  (via drill 0.2)
  Top 0.127: U3.13 v8.8,23.01
  Horz 0.127: v3.5,23.01 3.5,23.09 3.66,23.25 8.6,23.25 8.8,23.05 v8.8,23.01 | v2.94,8.89 3.12,8.89 4.43,7.58 v6.8,7.58
  Vert 0.127: v3.5,23.01 3.1,22.61 3.1,9.05 v2.94,8.89
  Bottom 0.127: J1.68 3.5,6.97 2.94,7.53 v2.94,8.89 | J1.56 6.5,7.28 v6.8,7.58
SPI_!CS1!/SDIO_DAT3/RX2  (via drill 0.2)
  Top 0.127: U3.12 v9.2,23.41
  Horz 0.127: v9.2,23.41 9.16,23.41 9.09,23.48 3.06,23.48 v3,23.42 v3,23.41 | v15.33,9.51 15.15,9.33 2.8,9.33 2.5,9.03 v2.5,8.71
  Vert 0.127: v3,23.41 2.5,22.91 v2.5,8.71
  Bottom 0.127: J1.70 3,7.04 2.5,7.54 v2.5,8.71 | J1.20 15.5,8.8 15.33,8.97 v15.33,9.51
SPI_!CS!/G5  (via drill 0.2)
  Top 0.127: J1.73 2.25,6.99 2.05,7.19 2.05,8.86 3.2,10.01 5.82,10.01 v5.82,10.04 5.84,10.02 8.11,10.02 9.51,11.41 9.51,12.02 9.6,12.11 U3.32 | J1.55 6.75,6.87 7.22,7.34 7.22,7.91 v7.12,8.01
  Bottom 0.127: v5.82,10.04 6.58,9.27 6.58,8.24 6.8,8.01 v7.12,8.01
SPI_CIPO1/SDIO_DAT0  (via drill 0.2)
  Top 0.127: U3.15 6.5,18.71 6.2,19.01 v4.2,19.01
  Vert 0.127: v4.2,19.01 4.2,11.63 4.12,11.55 4.12,10.99 v4.3,10.81
  Bottom 0.127: J1.64 4.5,6.93 4.32,7.11 4.32,10.79 v4.3,10.81
SPI_CIPO/G4  (via drill 0.2)
  Top 0.127: J1.61 5.25,7.83 v4.96,8.11 | U3.31 9.2,11.55 8.64,10.99 7.68,10.99 7.6,10.91 7.6,10.61 7.66,10.55 v8.05,10.55
  Horz 0.127: v8.05,10.55 7.82,10.55 6.95,11.43 5.67,11.43 5.14,10.9 v5.14,10.61
  Vert 0.127: v5.14,10.61 5.14,8.29 v4.96,8.11
  Bottom 0.127: J1.48 8.5,7.41 8.89,7.8 8.89,8.32 7.98,9.23 7.07,9.23 6.99,9.31 6.99,9.5 7.1,9.61 8.08,9.61 8.18,9.71 8.18,10.01 8.08,10.11 7.1,10.11 6.99,10.22 6.99,10.61 7.08,10.71 7.91,10.71 v8.05,10.55
SPI_COPI1/SDIO_CMD  (via drill 0.2)
  Top 0.127: U3.18 5.26,17.51 v4.76,18.01
  Vert 0.127: v4.76,18.01 4.46,17.71 v4.46,11.41
  Bottom 0.127: v4.46,11.41 4.64,11.23 4.64,8.38 4.55,8.28 4.55,7.86 5.14,7.27 5.14,6.97 5,6.83 J1.62
SPI_COPI/G7  (via drill 0.2)
  Top 0.127: U3.35 10.8,11.18 9.03,9.41 7.8,9.41 v7.01,8.61 v7,8.61 | J1.69 3.25,6.22 3.15,6.32 3.15,8.06 3.58,8.49 4.76,8.49 4.79,8.53 5.14,8.53 5.36,8.31 v5.8,8.31 5.75,8.26 J1.59
  Horz 0.127: v5.8,8.31 6.1,8.61 v7,8.61
SPI_SCK1/SDIO_CLK  (via drill 0.2)
  Top 0.127: U3.17 v5.9,17.91
  Vert 0.127: v5.9,17.91 5.5,17.51 5.5,10.87 5.91,10.46 5.99,10.46 6.24,10.21 6.24,9.87 5.61,9.24 v5.61,8.81
  Bottom 0.127: J1.60 5.5,8.02 5.38,8.14 5.38,8.48 5.61,8.71 v5.61,8.81
SPI_SCK/G6
  Top 0.127: U3.34 10.4,11.21 8.9,9.71 7.08,9.71 6.99,9.62 6.3,9.62 | 6.3,9.62 3.98,9.62 3.8,9.44 3.8,9.01 3.6,8.81 3.47,8.81 2.75,8.09 J1.71 | J1.57 6.25,9.57 6.3,9.62
SWDCK  (via drill 0.2)
  Top 0.127: v15.3,10.51 15.25,10.46 15.25,9.91 14.99,9.65 14.99,9.37 15.25,9.11 J1.21 | v5.84,11.01 5.84,11.51 5.43,11.92 5.43,14.74 5.8,15.11 U3.24
  Horz 0.127: v15.3,10.51 12.4,10.51 12.03,10.14 7.71,10.14 6.78,11.06 5.89,11.06 v5.84,11.01
SWDIO  (via drill 0.2)
  Top 0.127: J1.23 14.75,10.1 v14.8,10.15 | U3.25 5.9,14.71 5.66,14.47 5.66,12.1 6.34,11.42 v6.34,10.62
  Horz 0.127: v14.8,10.15 12.37,10.15 12.12,9.91 7.55,9.91 6.84,10.62 v6.34,10.62
TX1  (via drill 0.2)
  Top 0.127: U3.2 v13.2,21.41 | J1.17 16.25,8.96 16.47,9.19 v16.47,9.69
  Horz 0.127: v16.5,21.61 15.18,21.61 14.84,21.27 14.56,21.27 14.42,21.41 v13.2,21.41
  Vert 0.127: v16.47,9.69 16.32,9.84 16.32,12.21 16.33,12.21 16.33,21.44 v16.5,21.61
USB_D+  (via drill 0.2)
  Top 0.127: J1.3 19.75,14.76 19,15.51 v19,17.21
  Bottom 0.127: v19,17.21 U2.3
USB_D-  (via drill 0.2)
  Top 0.127: J1.5 19.25,6.56 19.52,6.83 19.52,14.4 v19.21,14.71
  Bottom 0.127: U2.7 19.5,14.42 v19.21,14.71
USB_MUX_SIG
  Bottom 0.127: U2.1 18,17.61 R5.2 R18.2
USB_VIN  (via drill 0.2)
  Top 0.127: v21.2,18.11 21.1,18.01 18.6,18.01 18.16,17.57 18.16,13.91 18.16,9.25 18.36,9.05 18.36,8.77 18.13,8.54 18.13,6.45 18.25,6.34 J1.9
  Bottom 0.127: v21.2,18.11 R18.1
USBHOST_D+  (via drill 0.2)
  Top 0.127: J1.35 11.75,7.16 v11.24,7.67
  Horz 0.127: v18.5,13.77 17.4,12.67 13.84,12.67 12.6,13.91 v11.2,13.91
  Vert 0.127: v11.24,7.67 11.24,11.45 11.2,11.49 v11.2,13.91 | v18.57,17.4 18.57,13.84 v18.5,13.77
  Bottom 0.127: U2.2 18.5,17.33 v18.57,17.4
USBHOST_D-  (via drill 0.2)
  Top 0.127: J1.37 11.25,7.08 v11.24,7.09
  Horz 0.127: v10.75,14.01 10.86,13.9 10.86,13.77 11.06,13.57 12.62,13.57 13.75,12.44 17.5,12.44 18.48,13.43 18.64,13.43 18.92,13.71 19.4,13.71 19.6,13.51 19.6,12.91 19.4,12.71 v19,12.71
  Vert 0.127: v10.75,14.01 10.86,13.9 10.86,7.27 11.04,7.09 v11.24,7.09
  Bottom 0.127: v19,12.71 U2.8

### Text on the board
Bottom: v10
Dimension: Units in mm
tDocu: 0.8mm PCB / 45 degree chamfered edge / Four layer design | N. Seidle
